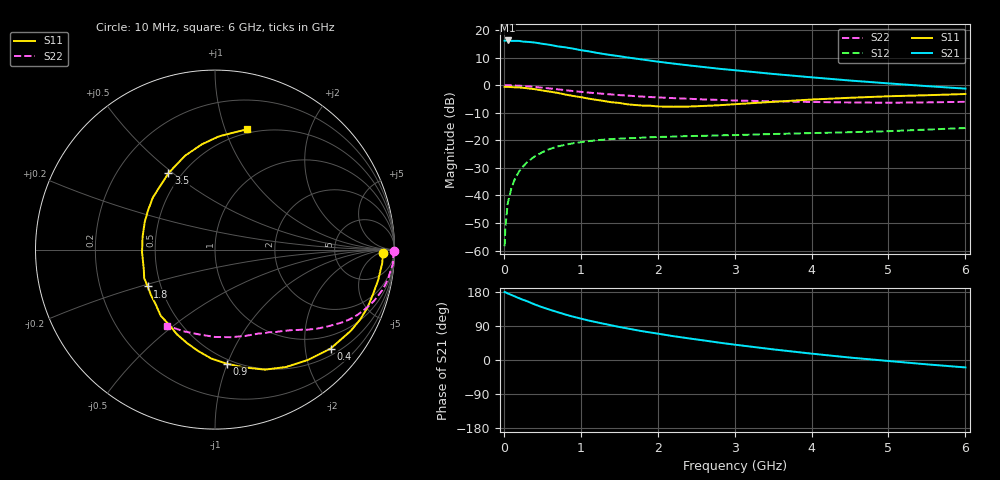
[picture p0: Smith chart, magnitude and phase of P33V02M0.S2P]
! SIEMENS Small Signal Semiconductors
! BFP181
! Si NPN RF Bipolar Junction Transistor in SOT143
! VCE = 3 V  IC = 2 mA
! Common Emitter S-Parameters:  March  1996
# GHz  S  MA  R  50
!  f  S11  S21  S12  S22
! GHz  MAG  ANG  MAG  ANG  MAG  ANG  MAG  ANG
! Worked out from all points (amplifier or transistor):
!   36 points, 10 MHz to 6 GHz, reference 50 ohm
!   highest |S21| = 16.2 dB at 50 MHz (marker M1)
!   |S21| within 3 dB of that: start of sweep to 906.9 MHz
!   unconditionally stable (mu >= 1): 2.465 GHz to end of sweep
!   at 250 MHz: K = 0.13, MSG = 22.7 dB, |S12| = -29.5 dB
!   at 1.4 GHz: K = 0.64, MSG = 15.2 dB, |S12| = -19.6 dB
!   at 6 GHz: K = 1.14, MAG = 4.9 dB, |S12| = -15.5 dB
!   lowest NFmin = 1.35 dB at 450 MHz
!   S11 on the Smith chart (normalised r, x): 10 MHz: 27, -8; 400 MHz: 0.65, -2.56; 900 MHz: 0.46, -0.99; 1.8 GHz: 0.42, -0.21; 3.5 GHz: 0.43, +0.48; 6 GHz: 0.46, +1.19
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0.01  0.9336 -1.2  6.421 179.3  0.0012 83.9  0.9968 -0.4
0.02  0.9358 -2.3  6.431 178.8  0.0026 87.0  0.9947 -1.0
0.05  0.9345 -4.8  6.489 175.7  0.0071 88.5  0.9937 -2.4
0.1  0.9248 -10.5  6.368 171.5  0.0139 82.2  0.9939 -4.8
0.2  0.9089 -20.8  6.358 162.9  0.0274 77.3  0.9789 -9.3
0.3  0.8817 -30.9  6.134 155.3  0.0397 71.6  0.9585 -13.7
0.4  0.8476 -40.6  5.955 146.7  0.051 66.0  0.9315 -17.8
0.5  0.8029 -50.1  5.648 139.2  0.0607 60.2  0.9016 -21.4
0.6  0.7641 -58.9  5.397 132.6  0.07 55.7  0.8726 -24.7
0.7  0.7248 -67.3  5.068 126.2  0.0773 51.6  0.8424 -27.6
0.8  0.6769 -76.0  4.866 120.0  0.0832 47.8  0.8134 -30.0
0.9  0.6387 -84.2  4.614 114.4  0.0883 44.3  0.7835 -32.3
1.1  0.5718 -99.7  4.125 104.3  0.0966 38.6  0.7353 -36.3
1.3  0.5174 -114.2  3.685 95.6  0.1028 34.1  0.6972 -39.5
1.5  0.4767 -129.4  3.363 87.2  0.1071 30.7  0.6619 -42.3
1.8  0.4277 -151.3  2.928 76.0  0.1118 27.0  0.6218 -46.1
2.2  0.4067 -178.0  2.471 63.0  0.1167 22.9  0.583 -51.3
2.8  0.433 149.2  1.988 45.8  0.123 19.0  0.5413 -59.5
3.5  0.4989 121.3  1.602 28.1  0.1301 16.4  0.5105 -70.3
4.5  0.5918 96.9  1.216 6.4  0.1403 12.9  0.4869 -89.9
5.5  0.6581 81.4  0.963 -11.5  0.1566 11.5  0.4878 -111.3
6  0.6927 75.2  0.867 -19.6  0.1671 9.6  0.5001 -122.2
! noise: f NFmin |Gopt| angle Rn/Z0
0.45  1.35  0.6  17  0.4
0.9  1.45  0.5  36  0.4
1.8  1.8  0.31  80  0.37
